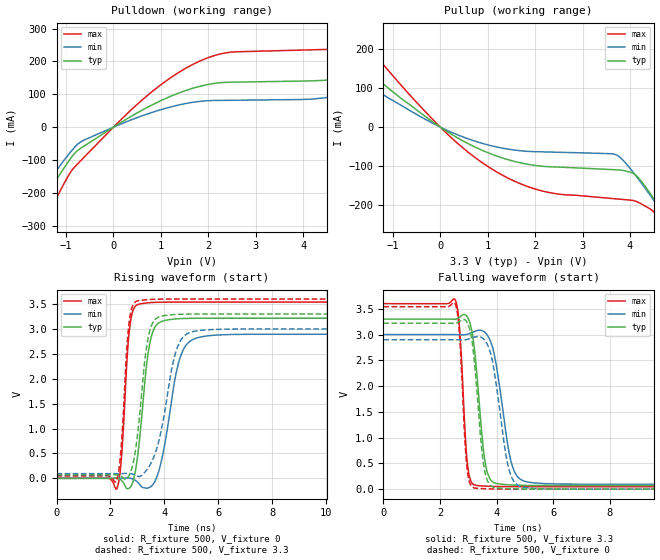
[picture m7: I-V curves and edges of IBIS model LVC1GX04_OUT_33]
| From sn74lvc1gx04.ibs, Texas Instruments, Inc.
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[Model]   LVC1GX04_OUT_33
Model_type  Output
Vref =   0
Rref =   500
Cref =   50p
Vmeas =   1.5
| variable   typ   min   max
C_comp   9.53pF   5.86pF   13.18pF
| C_pullup   9.86pF   5.86pF   11.98pF
| C_pulldown   9.20pF   6.49pF   13.18pF
[Temperature Range]   40   100   -40
| Ambient temperature   25   85   -40
[Voltage range]   3.3   3   3.6
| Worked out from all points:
|   slope of the pulldown table from 0 to 0.495 V, typ, clamps not added: 11.5 ohm
|   slope of the pullup table from 0 to 0.495 V, typ, clamps not added: 13.6 ohm
|   rising waveform, R_fixture 500, V_fixture 0: 20-80 % time 364ps typ, 547ps min, 230ps max; typ from 0 V to 3.22 V
|   falling waveform, R_fixture 500, V_fixture 3.3: 20-80 % time 314ps typ, 469ps min, 204ps max; typ from 3.3 V to 0.071 V
|   rising waveform, R_fixture 500, V_fixture 3.3: 20-80 % time 378ps typ, 606ps min, 232ps max; typ from 0.07 V to 3.3 V
|   falling waveform, R_fixture 500, V_fixture 0: 20-80 % time 305ps typ, 450ps min, 200ps max; typ from 3.22 V to 0 V
[Pulldown]
| LVC1GX04_OUT_33
|   Voltage   I(typ)   I(min)   I(max)
-5.5V     -1.107A    -970.8mA   -1.353A
-2.055V   -353.2mA   -300.4mA   -454.5mA
-1.49V    -224.6mA   -188.2mA   -296.4mA
-740mV    -69.5mA    -50.1mA    -109.7mA
365mV     32.28mA    21.63mA    51.56mA
2.22V     134.9mA    81.36mA    221.6mA
4.92V     153.7mA    101.9mA    243.5mA
6.98V     278.6mA    201.4mA    397.7mA
7.35V     308.4mA    129.2mA    438.3mA
7.84V     330.1mA    92.32mA    495.6mA
8.75V     170.7mA    93.06mA    502mA
11V       160mA      96.27mA    278.2mA
[Pullup]
| LVC1GX04_OUT_33
|   Voltage   I(typ)   I(min)   I(max)
-5.5V     609.5mA    479.2mA    854.2mA
-3.49V    364.8mA    283mA      516.7mA
-2.685V   271.1mA    208.6mA    386.5mA
-1.96V    190.3mA    144.9mA    273.3mA
-55mV     4.572mA    3.33mA     6.783mA
1.095V    -70.05mA   -48.34mA   -108.1mA
2.155V    -100.5mA   -63.45mA   -164.1mA
3.69V     -109.4mA   -70.27mA   -184mA
4.135V    -124.9mA   -126.7mA   -191mA
4.79V     -237.5mA   -238.3mA   -272mA
5V        -277.7mA   -275.7mA   -316.9mA
11V       -1.518A    -1.406A    -1.753A
[Ramp]
| LVC1GX04_OUT_33
| variable   typ   min   max
dV/dt_r   2.05/3.93E-10   1.86/5.92E-10   2.25/2.50E-10
dV/dt_f   1.99/3.30E-10   1.79/4.86E-10   2.19/2.19E-10
R_load = 500
[Rising Waveform]
| LVC1GX04_OUT_33
R_fixture =   500
C_fixture =   0
L_fixture =   0
V_fixture =   0
V_fixture_min = 0
V_fixture_max = 0
|   Time   V(typ)   V(min)   V(max)
0s        144.1pV    5.487nV    2.182nV
2.24ns    2.538mV    -42.86uV   -202.9mV
2.405ns   -37.69mV   864.7uV    393.3mV
2.72ns    -186.5mV   2.694mV    3.051V
3.06ns    682.2mV    -108mV     3.498V
3.36ns    2.364V     -198.4mV   3.523V
3.605ns   2.988V     -102.5mV   3.533V
4.57ns    3.207V     2.399V     3.539V
5.285ns   3.215V     2.832V     3.539V
24.99ns   3.216V     2.894V     3.539V
[Falling Waveform]
| LVC1GX04_OUT_33
R_fixture =   500
C_fixture =   0
L_fixture =   0
V_fixture =   3.3
V_fixture_min = 3
V_fixture_max = 3.6
|   Time   V(typ)   V(min)   V(max)
0s        3.3V       3V         3.6V
2.54ns    3.298V     2.999V     3.671V
2.695ns   3.339V     2.997V     3.092V
2.96ns    3.346V     3.004V     528.7mV
3.22ns    2.7V       3.06V      80.02mV
3.525ns   799.1mV    3.067V     62.01mV
3.695ns   284.1mV    2.967V     56.91mV
4.51ns    82.03mV    534.6mV    49.37mV
5.025ns   74.15mV    147.5mV    48.72mV
24.99ns   70.51mV    94.57mV    48.42mV
[Rising Waveform]
| LVC1GX04_OUT_33
R_fixture =   500
C_fixture =   0
L_fixture =   0
V_fixture =   3.3
V_fixture_min = 3
V_fixture_max = 3.6
|   Time   V(typ)   V(min)   V(max)
0s        70.47mV    94.51mV    48.4mV
2.215ns   74.43mV    94.43mV    -61.71mV
2.39ns    44.02mV    95.25mV    572.4mV
2.68ns    46.81mV    100mV      3.067V
2.975ns   739.6mV    51.26mV    3.559V
3.3ns     2.477V     138.2mV    3.585V
3.53ns    3.08V      331.4mV    3.594V
4.435ns   3.291V     2.553V     3.6V
5.065ns   3.299V     2.947V     3.6V
24.99ns   3.3V       3V         3.6V
[Falling Waveform]
| LVC1GX04_OUT_33
R_fixture =   500
C_fixture =   0
L_fixture =   0
V_fixture =   0
V_fixture_min = 0
V_fixture_max = 0
|   Time   V(typ)   V(min)   V(max)
0s        3.22V      2.9V       3.542V
2.535ns   3.218V     2.9V       3.598V
2.685ns   3.253V     2.897V     3.021V
2.945ns   3.247V     2.903V     457.4mV
3.21ns    2.497V     2.95V      22.23mV
3.48ns    745.3mV    2.939V     11.7mV
3.665ns   177.5mV    2.815V     7.181mV
4.415ns   9.619mV    426.6mV    976.4uV
4.91ns    3.052mV    41.21mV    336.6uV
24.99ns   37.16uV    51.83uV    25.27uV
